(* Logix 5000 Rung export; software revision 16.04 *)

MODULES
   MVI69MNET : vendor None type None code None
   Local : vendor None type None code None
END_MODULES

TYPE MNETCoilArray :   // Conversion to INT Values
STRUCT
   Boolean : BOOL[416];   // Description from B
END_STRUCT
END_TYPE

TYPE MNETConnectionOutput :
STRUCT
   Data : INT[61];
END_STRUCT
END_TYPE

TYPE MNETCONTROL :
STRUCT
   BootTimer : TIMER;
   ColdBoot : BOOL;
   WarmBoot : BOOL;
   ResetStatus : BOOL;   // Reset Status
   EventCmd : MNETEventCmd;
   CmdControl : MNETCmdControl;
   PassThru : MNETPassThru;
END_STRUCT
END_TYPE

TYPE MNETPortStats :   // This object is used to store the port statistics for an MVI69-MNet port.
STRUCT
   CmdReq : INT;   // Total number of command list requests sent
   CmdResp : INT;   // Total number of command list responses received
   CmdErr : INT;   // Total number of command list errors
   Requests : INT;   // Total number of requests for port
   Responses : INT;   // Total number of responses for port
   ErrSent : INT;   // Total number of errors sent
   ErrRec : INT;   // Total number of errors received
   CfgErrWord : INT;   // Configuration Error Word
   CurErr : INT;   // Current Error code
   LastErr : INT;   // Last recorded error code
END_STRUCT
END_TYPE

TYPE MNETEventCmd :
STRUCT
   EventCmdTrigger : BOOL;
   EventCmdPending : BOOL;
   IPaddress : INT[4];
   ServicePort : INT;
   NodeAddress : INT;
   InternalAddress : INT;
   Count : INT;
   Swap : INT;
   FunctionCode : INT;
   DeviceDBaddress : INT;
   EventCmdStatusReturned : INT;
   EventBlockID : INT;
END_STRUCT
END_TYPE

TYPE MNETCmdControl :
STRUCT
   CmdControlTrigger : BOOL;
   CmdControlPending : BOOL;
   CommandIndex : INT[6];
   CmdsAddedToQueue : INT;
   NumberOfCommands : INT;
   CmdControlBlockID : INT;
END_STRUCT
END_TYPE

TYPE MNETPassThru :
STRUCT
   MBControl1 : CONTROL;
   MBControl2 : CONTROL;
   MBOffsetByte : INT;
   MBOffsetBit : DINT;
   MBMsgLen : INT;
   MBMsg : SINT[500];
   MBScratch : INT[3];
   ByteLength : INT;
   MBMaskedVal : DINT;
   MBWordAddress : DINT;
   MBBitAddress : DINT;
   MBdouble : DINT;
   MBCoil : MNETCoilArray;
END_STRUCT
END_TYPE

TYPE MNETModuleDef :
STRUCT
   CONFIG : MNETCONFIG;
   DATA : MNETDATA;
   STATUS : MNETSTATUS;   // Status information in each read block
   CONTROL : MNETCONTROL;
   UTIL : MNETUTIL;
END_STRUCT
END_TYPE

TYPE MNETCONFIG :
STRUCT
   BlockTransferSize : INT;
END_STRUCT
END_TYPE

TYPE MNETConnectionInput :
STRUCT
   Data : INT[62];
END_STRUCT
END_TYPE

TYPE MNETBlockStats :   // This object is used to store the block transfer statistics for the MVI69-MNet module.
STRUCT
   Read : INT;   // Total number of read block transfers
   Write : INT;   // Total number of write block transfers
   Parse : INT;   // Total number of blocks parsed
   Event : INT;   // Total number of event blocks received
   Cmd : INT;   // Total number of command blocks received
   Err : INT;   // Total number of block transfer errors
END_STRUCT
END_TYPE

TYPE MNETSTATUS :   // This status data is returned on each read block and can be used to detect proper module operation.
STRUCT
   PassCnt : INT;   // Program cycle counter
   Block : MNETBlockStats;   // Block transfer statistics
   MnetServer : MNETPortStats;   // MNet server status data
   MBAPServer : MNETPortStats;   // MBAP server status data
   ClientStatus : MNETPortStats;   // Client status data
END_STRUCT
END_TYPE

TYPE MNETUTIL :
STRUCT
   ReadDataSizeGet : INT;   // Gets ReadData Array Length.
   WriteDataSizeGet : INT;   // Gets WriteData Array Length.
   ReadDataBlkCount : INT;   // holds the value of the Block Counts of the Read Data Array.
   WriteDataBlkCount : INT;   // holds the value of the Block Counts of the Write Data Array.
   RBTSremainder : INT;   // The remainder of the 60, 120 or 240 block to transfer.
   WBTSremainder : INT;   // The remainder of the 60, 120 or 240 block to transfer.
   LastRead : INT;
   LastWrite : INT;
   BlockIndex : INT;
END_STRUCT
END_TYPE

TYPE MNETDATA :
STRUCT
   ReadData : INT[600];
   WriteData : INT[600];
END_STRUCT
END_TYPE

ADD_ON_INSTRUCTION AOI69MNET   (* revision 1.6, vendor ProSoft Technology Inc. *)
// Add On instruction interface between the CompactLogix backplane and the MVI69-MNET module.
// Revision note:
// v1.6 - Changed Block 9958 function to avoid Minor Overflow Fault occurring on bit16 of every word transmitted from WriteData[ ]
// Help:
// v1.6 - Changed Block 9958 function to avoid Minor Overflow Fault occurring on bit16 of every word transmitted from WriteData[ ]
// v1.4 - Added Block 9997 function to reset status
// No Add-On functionality change.
// The revision level was updated to reflect the rung import change  which replaced the COP instruction by CPS for data integrity.
VAR_IN_OUT
   Connection_Input : MNETConnectionInput; {required}
   Connection_Output : MNETConnectionOutput; {required}
   MNET : MNETModuleDef; {required}
END_VAR

ROUTINE Logic   (* ladder *)
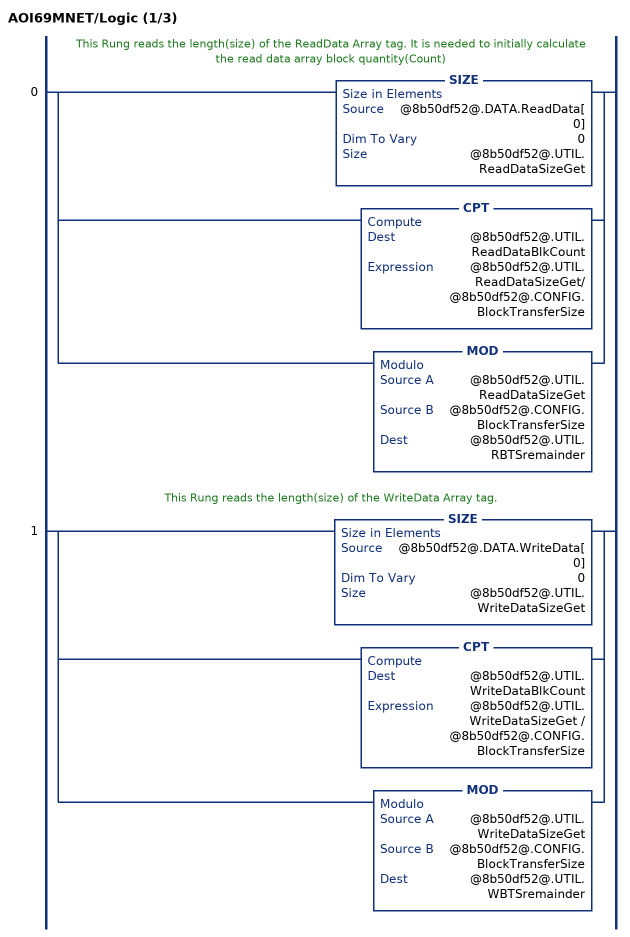
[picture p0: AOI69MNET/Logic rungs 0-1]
   // This Rung reads the length(size) of the ReadData Array tag. It is needed to initially calculate the read data array block quantity(Count)
   0: [SIZE(@8b50df52@.DATA.ReadData[0],0,@8b50df52@.UTIL.ReadDataSizeGet) ,CPT(@8b50df52@.UTIL.ReadDataBlkCount,@8b50df52@.UTIL.ReadDataSizeGet/@8b50df52@.CONFIG.BlockTransferSize) ,MOD(@8b50df52@.UTIL.ReadDataSizeGet,@8b50df52@.CONFIG.BlockTransferSize,@8b50df52@.UTIL.RBTSremainder) ];
   // This Rung reads the length(size) of the WriteData Array tag.
   1: [SIZE(@8b50df52@.DATA.WriteData[0],0,@8b50df52@.UTIL.WriteDataSizeGet) ,CPT(@8b50df52@.UTIL.WriteDataBlkCount,@8b50df52@.UTIL.WriteDataSizeGet / @8b50df52@.CONFIG.BlockTransferSize) ,MOD(@8b50df52@.UTIL.WriteDataSizeGet,@8b50df52@.CONFIG.BlockTransferSize,@8b50df52@.UTIL.WBTSremainder) ];
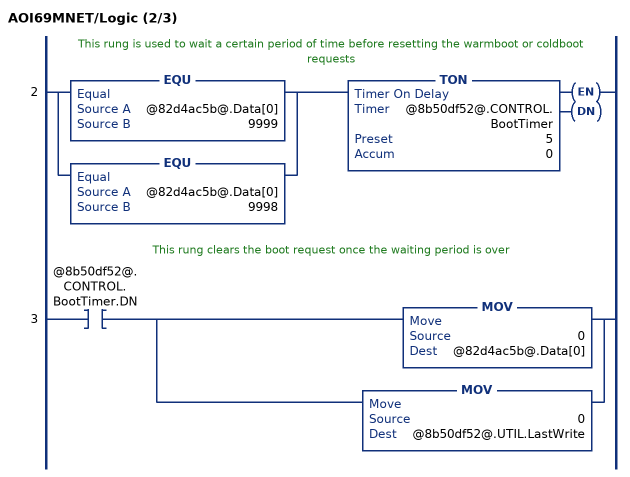
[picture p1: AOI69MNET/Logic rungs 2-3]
   // This rung is used to wait a certain period of time before resetting the warmboot or coldboot requests
   2: [EQU(@82d4ac5b@.Data[0],9999) ,EQU(@82d4ac5b@.Data[0],9998) ]TON(@8b50df52@.CONTROL.BootTimer,5,0);
   // This rung clears the boot request once the waiting period is over
   3: XIC(@8b50df52@.CONTROL.BootTimer.DN)[MOV(0,@82d4ac5b@.Data[0]) ,MOV(0,@8b50df52@.UTIL.LastWrite) ];
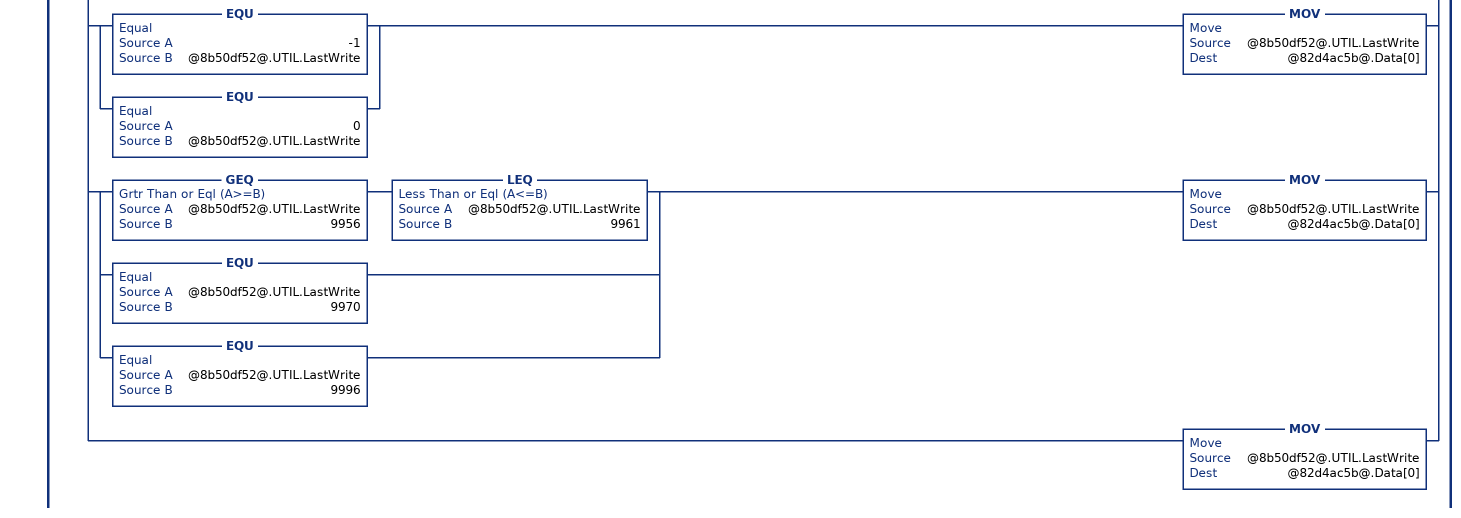
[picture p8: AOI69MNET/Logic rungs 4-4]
   // The routines will only be scanned once the processor receives a new read block ID from the module
   4: NEQ(@8b50df52@.UTIL.LastRead,@74053cb8@.Data[0])[MOV(@74053cb8@.Data[0],@8b50df52@.UTIL.LastRead) ,GEQ(@8b50df52@.UTIL.LastRead,1) [LEQ(@8b50df52@.UTIL.LastRead,@8b50df52@.UTIL.ReadDataBlkCount) [CPT(@8b50df52@.UTIL.BlockIndex,(@8b50df52@.UTIL.LastRead - 1) * @8b50df52@.CONFIG.BlockTransferSize) ,COP(@74053cb8@.Data[2],@8b50df52@.DATA.ReadData[@8b50df52@.UTIL.BlockIndex],@8b50df52@.CONFIG.BlockTransferSize) ] ,CMP(@8b50df52@.UTIL.LastRead - @8b50df52@.UTIL.ReadDataBlkCount = 1) GRT(@8b50df52@.UTIL.RBTSremainder,0) [CPT(@8b50df52@.UTIL.BlockIndex,(@8b50df52@.UTIL.LastRead - 1) * @8b50df52@.CONFIG.BlockTransferSize) ,COP(@74053cb8@.Data[2],@8b50df52@.DATA.ReadData[@8b50df52@.UTIL.BlockIndex],@8b50df52@.UTIL.RBTSremainder) ] ] ,[EQU(@8b50df52@.UTIL.LastRead,-1) ,EQU(@8b50df52@.UTIL.LastRead,0) ] [COP(@74053cb8@.Data[2],@8b50df52@.STATUS.PassCnt,1) ,COP(@74053cb8@.Data[3],@8b50df52@.STATUS.Block.Read,6) ,COP(@74053cb8@.Data[19],@8b50df52@.STATUS.MnetServer.CmdReq,10) ,COP(@74053cb8@.Data[29],@8b50df52@.STATUS.MBAPServer.CmdReq,10) ,COP(@74053cb8@.Data[39],@8b50df52@.STATUS.ClientStatus.CmdReq,10) ] ,EQU(@8b50df52@.UTIL.LastRead,2000) [MOV(@8b50df52@.UTIL.LastRead,@8b50df52@.CONTROL.EventCmd.EventBlockID) ,MOV(@74053cb8@.Data[2],@8b50df52@.CONTROL.EventCmd.EventCmdStatusReturned) ,OTU(@8b50df52@.CONTROL.EventCmd.EventCmdPending) ,OTU(@8b50df52@.CONTROL.EventCmd.EventCmdTrigger) ] ,LIM(5001,@8b50df52@.UTIL.LastRead,5006) [MOV(@8b50df52@.UTIL.LastRead,@8b50df52@.CONTROL.CmdControl.CmdControlBlockID) ,MOV(@74053cb8@.Data[2],@8b50df52@.CONTROL.CmdControl.CmdsAddedToQueue) ,OTU(@8b50df52@.CONTROL.CmdControl.CmdControlPending) ,OTU(@8b50df52@.CONTROL.CmdControl.CmdControlTrigger) ] ,EQU(9996,@8b50df52@.UTIL.LastRead) [MOV(@74053cb8@.Data[2],@8b50df52@.CONTROL.PassThru.MBMsgLen) ,COP(@74053cb8@.Data[3],@8b50df52@.CONTROL.PassThru.MBMsg[0],@8b50df52@.CONTROL.PassThru.MBMsgLen) ] ,LIM(9956,@8b50df52@.UTIL.LastRead,9957) LES(@74053cb8@.Data[3],600) [MOV(@74053cb8@.Data[3],@8b50df52@.CONTROL.PassThru.MBOffsetByte) ,COP(@74053cb8@.Data[4],@8b50df52@.DATA.WriteData[@8b50df52@.CONTROL.PassThru.MBOffsetByte],@74053cb8@.Data[2]) ] ,EQU(9958,@8b50df52@.UTIL.LastRead) MVM(@74053cb8@.Data[3],16#0000FFFF,@8b50df52@.CONTROL.PassThru.MBMaskedVal) LES(@8b50df52@.CONTROL.PassThru.MBMaskedVal,65535) [DIV(@8b50df52@.CONTROL.PassThru.MBMaskedVal,16,@8b50df52@.CONTROL.PassThru.MBWordAddress) MOD(@8b50df52@.CONTROL.PassThru.MBMaskedVal,16,@8b50df52@.CONTROL.PassThru.MBBitAddress) ,MOV(@74053cb8@.Data[4],@8b50df52@.CONTROL.PassThru.MBScratch[2]) ,NEQ(@8b50df52@.CONTROL.PassThru.MBScratch[2],0) OTL(@8b50df52@.DATA.WriteData[@8b50df52@.CONTROL.PassThru.MBWordAddress].[@8b50df52@.CONTROL.PassThru.MBBitAddress]) ,EQU(@8b50df52@.CONTROL.PassThru.MBScratch[2],0) OTU(@8b50df52@.DATA.WriteData[@8b50df52@.CONTROL.PassThru.MBWordAddress].[@8b50df52@.CONTROL.PassThru.MBBitAddress]) ] ,EQU(9959,@8b50df52@.UTIL.LastRead) [MOV(@74053cb8@.Data[3],@8b50df52@.CONTROL.PassThru.MBOffsetByte) ,MOV(@74053cb8@.Data[2],@8b50df52@.CONTROL.PassThru.MBControl1.LEN) ,MOV(@74053cb8@.Data[2],@8b50df52@.CONTROL.PassThru.MBControl2.LEN) ,FAL(@8b50df52@.CONTROL.PassThru.MBControl1,10,0,ALL,@8b50df52@.DATA.WriteData[@8b50df52@.CONTROL.PassThru.MBOffsetByte+@8b50df52@.CONTROL.PassThru.MBControl1.POS],@8b50df52@.DATA.WriteData[@8b50df52@.CONTROL.PassThru.MBOffsetByte+@8b50df52@.CONTROL.PassThru.MBControl1.POS] AND(NOT @74053cb8@.Data[34+@8b50df52@.CONTROL.PassThru.MBControl1.POS])) ,FAL(@8b50df52@.CONTROL.PassThru.MBControl2,10,0,ALL,@8b50df52@.DATA.WriteData[@8b50df52@.CONTROL.PassThru.MBOffsetByte+@8b50df52@.CONTROL.PassThru.MBControl2.POS],@8b50df52@.DATA.WriteData[@8b50df52@.CONTROL.PassThru.MBOffsetByte+@8b50df52@.CONTROL.PassThru.MBControl2.POS] OR(@74053cb8@.Data[4+@8b50df52@.CONTROL.PassThru.MBControl2.POS] AND @74053cb8@.Data[4+@8b50df52@.CONTROL.PassThru.MBControl2.POS])) ] ,EQU(9961,@8b50df52@.UTIL.LastRead) [MOV(@74053cb8@.Data[2],@8b50df52@.CONTROL.PassThru.MBMsgLen) ,CPT(@8b50df52@.CONTROL.PassThru.MBMsgLen,@8b50df52@.CONTROL.PassThru.MBMsgLen * 2 + 2) ,COP(@74053cb8@.Data[3],@8b50df52@.CONTROL.PassThru.MBMsg[0],@8b50df52@.CONTROL.PassThru.MBMsgLen) ] ,MOV(@74053cb8@.Data[1],@8b50df52@.UTIL.LastWrite) ,XIC(@8b50df52@.CONTROL.ColdBoot) [NEQ(@8b50df52@.UTIL.LastWrite,9999) ,NEQ(@82d4ac5b@.Data[0],9999) ] [MOV(9999,@8b50df52@.UTIL.LastWrite) ,OTU(@8b50df52@.CONTROL.ColdBoot) ] ,XIC(@8b50df52@.CONTROL.WarmBoot) [MOV(9998,@8b50df52@.UTIL.LastWrite) ,OTU(@8b50df52@.CONTROL.WarmBoot) ] ,XIC(@8b50df52@.CONTROL.ResetStatus) [MOV(9997,@8b50df52@.UTIL.LastWrite) ,OTU(@8b50df52@.CONTROL.ResetStatus) ] ,GEQ(@8b50df52@.UTIL.LastWrite,1) [LEQ(@8b50df52@.UTIL.LastWrite,@8b50df52@.UTIL.WriteDataBlkCount) [CPT(@8b50df52@.UTIL.BlockIndex,(@8b50df52@.UTIL.LastWrite - 1) * @8b50df52@.CONFIG.BlockTransferSize) ,COP(@8b50df52@.DATA.WriteData[@8b50df52@.UTIL.BlockIndex],@82d4ac5b@.Data[1],@8b50df52@.CONFIG.BlockTransferSize) ] ,CMP(@8b50df52@.UTIL.LastWrite - @8b50df52@.UTIL.WriteDataBlkCount = 1) GRT(@8b50df52@.UTIL.WBTSremainder,0) [CPT(@8b50df52@.UTIL.BlockIndex,(@8b50df52@.UTIL.LastWrite-1)*@8b50df52@.CONFIG.BlockTransferSize) ,COP(@8b50df52@.DATA.WriteData[@8b50df52@.UTIL.BlockIndex],@82d4ac5b@.Data[1],@8b50df52@.UTIL.WBTSremainder) ] ] ,LIM(1000,@8b50df52@.UTIL.LastWrite,1083) [CPT(@8b50df52@.UTIL.BlockIndex,(@8b50df52@.UTIL.LastWrite - 1000) * @8b50df52@.CONFIG.BlockTransferSize) ,COP(@8b50df52@.DATA.ReadData[@8b50df52@.UTIL.BlockIndex],@82d4ac5b@.Data[1],@8b50df52@.CONFIG.BlockTransferSize) ] ,XIC(@8b50df52@.CONTROL.EventCmd.EventCmdTrigger) XIO(@8b50df52@.CONTROL.EventCmd.EventCmdPending) [COP(@8b50df52@.CONTROL.EventCmd.IPaddress[0],@82d4ac5b@.Data[1],11) ,MOV(2000,@8b50df52@.UTIL.LastWrite) ,OTL(@8b50df52@.CONTROL.EventCmd.EventCmdPending) ] ,XIC(@8b50df52@.CONTROL.CmdControl.CmdControlTrigger) XIO(@8b50df52@.CONTROL.CmdControl.CmdControlPending) [COP(@8b50df52@.CONTROL.CmdControl.CommandIndex[0],@82d4ac5b@.Data[1],6) ,LIM(1,@8b50df52@.CONTROL.CmdControl.NumberOfCommands,6) ADD(5000,@8b50df52@.CONTROL.CmdControl.NumberOfCommands,@8b50df52@.UTIL.LastWrite) ,OTL(@8b50df52@.CONTROL.CmdControl.CmdControlPending) ] ,[EQU(-1,@8b50df52@.UTIL.LastWrite) ,EQU(0,@8b50df52@.UTIL.LastWrite) ] MOV(@8b50df52@.UTIL.LastWrite,@82d4ac5b@.Data[0]) ,[GEQ(@8b50df52@.UTIL.LastWrite,9956) LEQ(@8b50df52@.UTIL.LastWrite,9961) ,EQU(@8b50df52@.UTIL.LastWrite,9970) ,EQU(@8b50df52@.UTIL.LastWrite,9996) ] MOV(@8b50df52@.UTIL.LastWrite,@82d4ac5b@.Data[0]) ,MOV(@8b50df52@.UTIL.LastWrite,@82d4ac5b@.Data[0]) ];
END_ROUTINE
END_ADD_ON_INSTRUCTION

VAR_GLOBAL   (* controller tags *)
   MNET : MNETModuleDef;
   Connection_Input : MNETConnectionInput;
   Local:1:I : AB:1769_MODULE_INT_128Bytes:I:0;
   Local:1:O : AB:1769_MODULE_INT_122Bytes:O:0;
   Connection_Output : MNETConnectionOutput;
   AOI69MNET : AOI69MNET;
END_VAR

PROGRAM MainProgram

ROUTINE MainRoutine   (* ladder *)
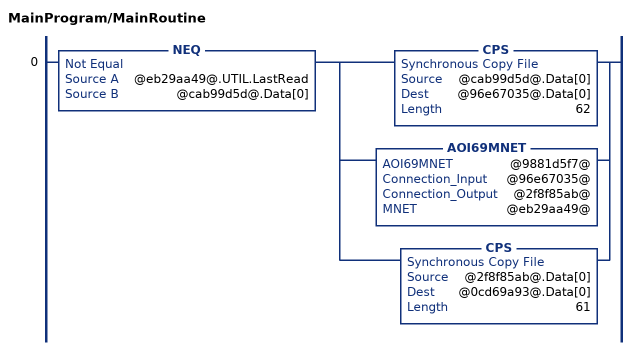
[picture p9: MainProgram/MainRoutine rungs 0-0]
   0: NEQ(@eb29aa49@.UTIL.LastRead,@cab99d5d@.Data[0])[CPS(@cab99d5d@.Data[0],@96e67035@.Data[0],62) ,AOI69MNET(@9881d5f7@,@96e67035@,@2f8f85ab@,@eb29aa49@) ,CPS(@2f8f85ab@.Data[0],@0cd69a93@.Data[0],61) ];
END_ROUTINE
END_PROGRAM
